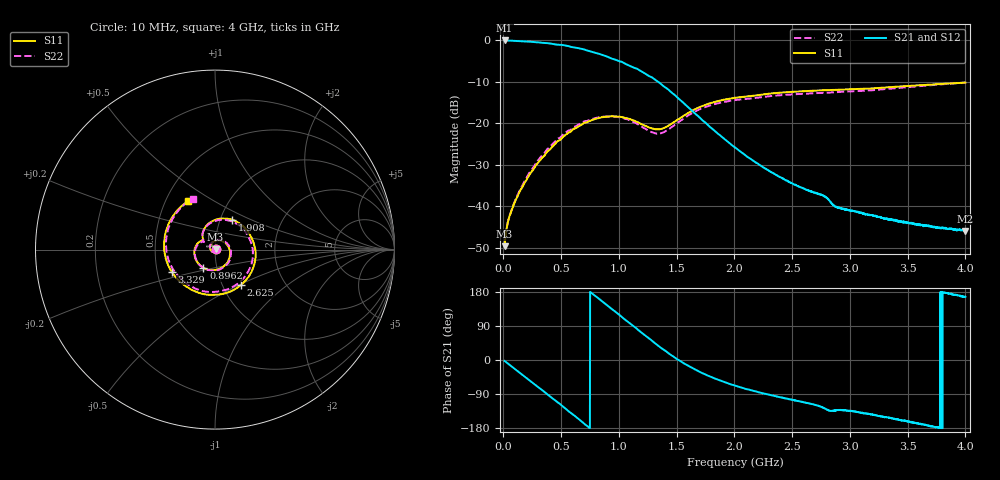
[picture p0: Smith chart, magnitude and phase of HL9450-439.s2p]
! 7/13/2020 7:51:30 AM
! H:\PRODUCTION_DATA\9450\10013\HL9450_10009_797MHZ_.S2P
! CHANNEL.1
! TR.MEASUREMENT
! CORRECTED.DATA
# GHZ S RI R 50.0
! FREQ.GHZ  S11RE  S11IM  S21RE  S21IM  S12RE  S12IM  S22RE  S22IM
!; PortSelection: Port_12
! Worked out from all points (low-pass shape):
!   2000 points, 10 MHz to 4 GHz, reference 50 ohm
!   highest |S21| = -0.03 dB at 10 MHz (marker M1); lowest = -46.0 dB at 3.994 GHz (marker M2)
!   |S21| within 3 dB of the highest: start of sweep to 796.4 MHz
!   lowest |S11| = -49.7 dB at 10 MHz (marker M3), VSWR 1.01, Z = 50.3 + j0.118 ohm
!   |S11| at or under -10 dB: start of sweep to end of sweep
!   |S22| runs from -49.6 to -10.2 dB; largest |S21 - S12| = 0.006
!   S11 on the Smith chart (normalised r, x): 10 MHz: 1.01, +0.00; 896.2 MHz: 0.86, -0.18; 1.908 GHz: 1.14, +0.39; 2.625 GHz: 1.22, -0.51; 3.329 GHz: 0.59, -0.16; 4 GHz: 0.65, +0.38
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0.01  0.00307 0.00117  0.9959 -0.0433  0.997 -0.0435  0.00307 0.00121
0.04991996  0.00666 -0.00313  0.9707 -0.2077  0.9709 -0.2079  0.00663 -0.00329
0.1197799  -0.00108 -0.0129  0.8627 -0.4728  0.8628 -0.4727  -0.00178 -0.0132
0.2415358  -0.0257 0.000732  0.5166 -0.8116  0.5168 -0.8103  -0.0273 0.0018
0.3533117  -0.0165 0.0369  0.1013 -0.9251  0.1014 -0.9251  -0.0173 0.04
0.5010155  0.0488 0.0422  -0.4291 -0.7712  -0.4282 -0.7706  0.0517 0.0458
0.6766633  0.0759 -0.0591  -0.7519 -0.2429  -0.7518 -0.2425  0.0816 -0.0589
0.8962231  -0.0644 -0.1009  -0.5185 0.3719  -0.5192 0.3702  -0.0609 -0.1044
1.067879  -0.1148 -0.00707  -0.1161 0.4973  -0.1131 0.4991  -0.1116 -0.0101
1.341331  -0.0653 0.0535  0.2494 0.1919  0.2498 0.1899  -0.0608 0.0435
1.57087  -0.0628 0.1085  0.167 -0.0306  0.167 -0.0302  -0.0682 0.0946
1.908194  0.0968 0.1658  0.0348 -0.0553  0.035 -0.0551  0.082 0.1605
2.005998  0.1493 0.1371  0.0195 -0.0471  0.0193 -0.0472  0.1342 0.135
2.321366  0.2267 -0.0304  -0.00144 -0.0255  -0.00144 -0.0256  0.2117 -0.0253
2.624757  0.1437 -0.1981  -0.00609 -0.0144  -0.00612 -0.0146  0.1305 -0.1865
2.670665  0.1199 -0.2153  -0.00664 -0.0134  -0.00662 -0.0133  0.107 -0.2028
2.896213  -0.016 -0.2523  -0.00646 -0.0071  -0.00647 -0.00713  -0.0249 -0.2364
3.329345  -0.242 -0.1226  -0.006 -0.00327  -0.00609 -0.00337  -0.2407 -0.0985
3.335333  -0.2441 -0.1194  -0.00609 -0.0033  -0.00618 -0.0033  -0.2422 -0.0948
3.652696  -0.2782 0.0812  -0.00569 -0.000964  -0.00577 -0.000885  -0.2633 0.1062
3.994012  -0.1561 0.2662  -0.0049 0.00114  -0.00496 0.00125  -0.1255 0.2825
4  -0.1527 0.2685  -0.00492 0.00116  -0.00492 0.00126  -0.1222 0.2844
